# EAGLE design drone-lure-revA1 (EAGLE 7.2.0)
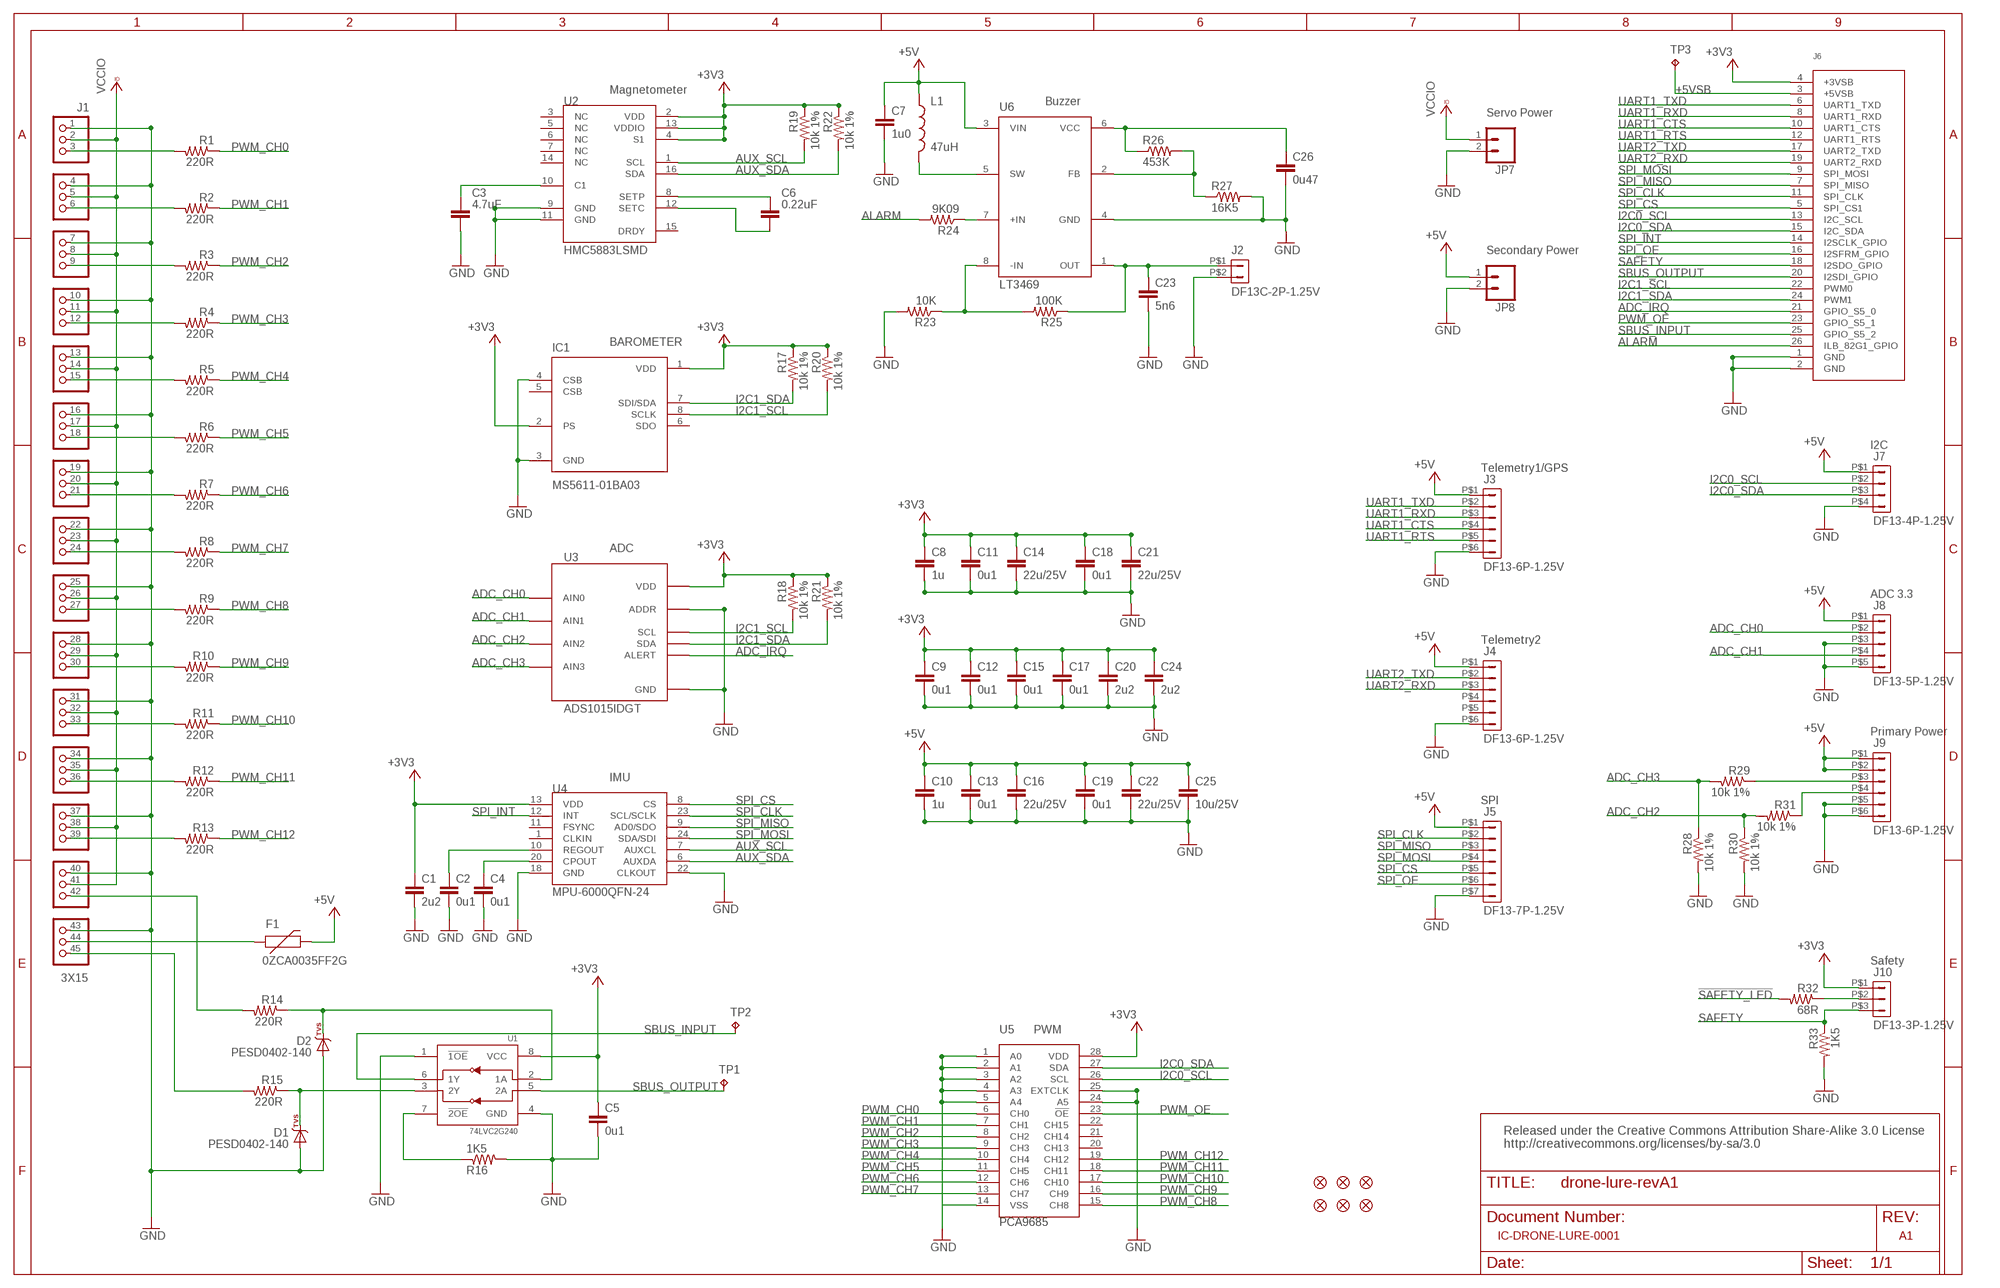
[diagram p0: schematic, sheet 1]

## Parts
C1  2u2  CAP0603  [0603-CAP]
C2  0u1  CAP0402  [0402-CAP]
C3  4.7uF  CAPACITOR_NPOL-0805  [C805]
C4  0u1  CAP0402  [0402-CAP]
C5  0u1  CAP0402  [0402-CAP]
C6  0.22uF  CAPACITOR_NPOL-0805  [C805]
C7  1u0  CAP0603  [0603-CAP]
C8  1u  CAP0603  [0603-CAP]
C9  0u1  CAP0402  [0402-CAP]
C10  1u  CAP0603  [0603-CAP]
C11  0u1  CAP0402  [0402-CAP]
C12  0u1  CAP0402  [0402-CAP]
C13  0u1  CAP0402  [0402-CAP]
C14  22u/25V  CAP0805  [0805-CAP]
C15  0u1  CAP0402  [0402-CAP]
C16  22u/25V  CAP0805  [0805-CAP]
C17  0u1  CAP0402  [0402-CAP]
C18  0u1  CAP0402  [0402-CAP]
C19  0u1  CAP0402  [0402-CAP]
C20  2u2  CAP0603  [0603-CAP]
C21  22u/25V  CAP0805  [0805-CAP]
C22  22u/25V  CAP0805  [0805-CAP]
C23  5n6  CAP0402  [0402-CAP]
C24  2u2  CAP0603  [0603-CAP]
C25  10u/25V  CAP0805  [0805-CAP]
C26  0u47  CAP0402  [0402-CAP]
D1  PESD0402-140  DIODE-TVS  [0402-TVS]
D2  PESD0402-140  DIODE-TVS  [0402-TVS]
F1  0ZCA0035FF2G  PTCSMD  [PTC-1206]
IC1  MS5611-01BA03  [SON125P300X500X100-8N]
J1  3X15  [3X15]
J2  DF13C-2P-1.25V  DF13-2P-1.25V  [DF13C-2P-1.25V]
J3  DF13-6P-1.25V  [DF13C-6P-1.25V]
J4  DF13-6P-1.25V  [DF13C-6P-1.25V]
J5  DF13-7P-1.25V  [DF13C-7P-1.25V]
J6  MBM_LOW_SPEED  [MBM_LOW_SPEED]
J7  DF13-4P-1.25V  [DF13C-4P-1.25V]
J8  DF13-5P-1.25V  [DF13C-5P-1.25V]
J9  DF13-6P-1.25V  [DF13C-6P-1.25V]
J10  DF13-3P-1.25V  [DF13C-3P-1.25V]
JP1  FIDUCIAL1X2.5  [FIDUCIAL-1X2.5]
JP2  FIDUCIAL1X2.5  [FIDUCIAL-1X2.5]
JP3  FIDUCIAL1X2.5  [FIDUCIAL-1X2.5]
JP4  FIDUCIAL1X2.5  [FIDUCIAL-1X2.5]
JP5  FIDUCIAL1X2.5  [FIDUCIAL-1X2.5]
JP6  FIDUCIAL1X2.5  [FIDUCIAL-1X2.5]
JP7  M023.5MM  [SCREWTERMINAL-3.5MM-2]
JP8  M023.5MM  [SCREWTERMINAL-3.5MM-2]
L1  47uH  INDUCTOR0805  [0805-IND]
R1  220R  RESISTOR0402-RES  [0402-RES]
R2  220R  RESISTOR0402-RES  [0402-RES]
R3  220R  RESISTOR0402-RES  [0402-RES]
R4  220R  RESISTOR0402-RES  [0402-RES]
R5  220R  RESISTOR0402-RES  [0402-RES]
R6  220R  RESISTOR0402-RES  [0402-RES]
R7  220R  RESISTOR0402-RES  [0402-RES]
R8  220R  RESISTOR0402-RES  [0402-RES]
R9  220R  RESISTOR0402-RES  [0402-RES]
R10  220R  RESISTOR0402-RES  [0402-RES]
R11  220R  RESISTOR0402-RES  [0402-RES]
R12  220R  RESISTOR0402-RES  [0402-RES]
R13  220R  RESISTOR0402-RES  [0402-RES]
R14  220R  RESISTOR0402-RES  [0402-RES]
R15  220R  RESISTOR0402-RES  [0402-RES]
R16  1K5  RESISTOR0402-RES  [0402-RES]
R17  10k 1%  RESISTOR0402-RES  [0402-RES]
R18  10k 1%  RESISTOR0402-RES  [0402-RES]
R19  10k 1%  RESISTOR0402-RES  [0402-RES]
R20  10k 1%  RESISTOR0402-RES  [0402-RES]
R21  10k 1%  RESISTOR0402-RES  [0402-RES]
R22  10k 1%  RESISTOR0402-RES  [0402-RES]
R23  10K  RESISTOR0402-RES  [0402-RES]
R24  9K09  RESISTOR0402-RES  [0402-RES]
R25  100K  RESISTOR0402-RES  [0402-RES]
R26  453K  RESISTOR0402-RES  [0402-RES]
R27  16K5  RESISTOR0402-RES  [0402-RES]
R28  10k 1%  RESISTOR0402-RES  [0402-RES]
R29  10k 1%  RESISTOR0402-RES  [0402-RES]
R30  10k 1%  RESISTOR0402-RES  [0402-RES]
R31  10k 1%  RESISTOR0402-RES  [0402-RES]
R32  68R  RESISTOR0402-RES  [0402-RES]
R33  1K5  RESISTOR0402-RES  [0402-RES]
TP1  TPTP07SQ  [TP07SQ]
TP2  TPTP07SQ  [TP07SQ]
TP3  TPTP15SQ  [TP15SQ]
U1  74LVC2G240  74LVC2G240-TSSOP-8  [TSSOP8_SOT505-2]
U2  HMC5883LSMD  [16LPCC]
U3  ADS1015IDGT  [MSOP10_0.5]
U4  MPU-6000QFN-24  [QFN-24-TESTING]
U5  PCA9685  [TSSOP-28_4MM]
U6  LT3469  [SOT23-8]

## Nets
!SAFETY_LED: R32.P$2
!SBUS_OUTPUT_EN: R16.P$1 U1.7(!2OE)
+3V3 [power]: C1.P$1 C5.P$1 C8.P$1 C9.P$1 C11.P$1 C12.P$1 C14.P$1 C15.P$1 C17.P$1 C18.P$1 C20.P$1 C21.P$1 C24.P$1 IC1.1(VDD) IC1.2(PS) J6.4(+3VSB) J10.P$1 R17.P$1 R18.P$1 R19.P$1 R20.P$1 R21.P$1 R22.P$1 U1.8(VCC) U2.2(VDD) U2.4(S1) U2.13(VDDIO) U3.8(VDD) U4.13(VDD) U5.28(VDD)
+5V [power]: C7.P$1 C10.P$1 C13.P$1 C16.P$1 C19.P$1 C22.P$1 C25.P$1 F1.2 J3.P$1 J4.P$1 J5.P$1 J7.P$1 J8.P$1 J9.P$1 J9.P$2 JP8.1 L1.P$1 U6.3(VIN)
+5VSB: J6.3(+5VSB) TP3.TP
ADC_CH0: J8.P$2 U3.4(AIN0)
ADC_CH1: J8.P$4 U3.5(AIN1)
ADC_CH2: R30.P$1 R31.P$2 U3.6(AIN2)
ADC_CH3: R28.P$1 R29.P$2 U3.7(AIN3)
ADC_IRQ: J6.21(GPIO_S5_0) U3.2(ALERT)
ALARM: J6.26(ILB_82G1_GPIO) R24.P$2
AUX_SCL: R19.P$2 U2.1(SCL) U4.7(AUXCL)
AUX_SDA: R22.P$2 U2.16(SDA) U4.6(AUXDA)
GND [power]: C1.P$2 C2.P$2 C3.2 C4.P$2 C5.P$2 C7.P$2 C8.P$2 C9.P$2 C10.P$2 C11.P$2 C12.P$2 C13.P$2 C14.P$2 C15.P$2 C16.P$2 C17.P$2 C18.P$2 C19.P$2 C20.P$2 C21.P$2 C22.P$2 C23.P$2 C24.P$2 C25.P$2 C26.P$2 D1.A D2.A IC1.3(GND) IC1.4(CSB) J1.1 J1.4 J1.7 J1.10 J1.13 J1.16 J1.19 J1.22 J1.25 J1.28 J1.31 J1.34 J1.37 J1.40 J1.43 J2.P$2 J3.P$6 J4.P$6 J5.P$7 J6.1(GND) J6.2(GND) J7.P$4 J8.P$3 J8.P$5 J9.P$5 J9.P$6 JP7.2 JP8.2 R16.P$2 R23.P$2 R27.P$2 R28.P$2 R30.P$2 R33.P$2 U1.1(!1OE) U1.4(GND) U2.9(GND) U2.11(GND) U3.1(ADDR) U3.3(GND) U4.18(GND) U4.22(CLKOUT) U5.1(A0) U5.2(A1) U5.3(A2) U5.4(A3) U5.5(A4) U5.14(VSS) U5.24(A5) U5.25(EXTCLK) U6.4(GND)
I2C0_SCL: J6.13(I2C_SCL) J7.P$2 U5.26(SCL)
I2C0_SDA: J6.15(I2C_SDA) J7.P$3 U5.27(SDA)
I2C1_SCL: IC1.8(SCLK) J6.22(PWM0) R18.P$2 R20.P$2 U3.10(SCL)
I2C1_SDA: IC1.7(SDI/SDA) J6.24(PWM1) R17.P$2 R21.P$2 U3.9(SDA)
N$1: C3.1 U2.10(C1)
N$2: J10.P$2 R32.P$1
N$3: C6.1 U2.8(SETP)
N$4: C6.2 U2.12(SETC)
N$5: J9.P$3 R29.P$1
N$6 [power]: F1.1 J1.44
N$7: J9.P$4 R31.P$1
N$8: J1.39 R13.P$2
N$9: J1.36 R12.P$2
N$10: J1.33 R11.P$2
N$11: J1.30 R10.P$2
N$12: J1.27 R9.P$2
N$13: J1.24 R8.P$2
N$14: J1.21 R7.P$2
N$15: J1.18 R6.P$2
N$16: J1.15 R5.P$2
N$17: J1.12 R4.P$2
N$18: J1.9 R3.P$2
N$19: J1.6 R2.P$2
N$20: J1.3 R1.P$2
N$21: R23.P$1 R25.P$2 U6.8(-IN)
N$23: C2.P$1 U4.10(REGOUT)
N$24: R26.P$2 R27.P$1 U6.2(FB)
N$25: C4.P$1 U4.20(CPOUT)
N$27 [power]: C23.P$1 J2.P$1 R25.P$1 U6.1(OUT)
N$28: R24.P$1 U6.7(+IN)
N$32: L1.P$2 U6.5(SW)
N$36 [power]: C26.P$1 R26.P$1 U6.6(VCC)
N$38: D1.C R15.P$1 U1.3(2Y)
PPM-SBUS-PROT [power]: J1.42 R14.P$2
PPM_INPUT: D2.C R14.P$1 U1.2(1A)
PWM_CH0: R1.P$1 U5.6(CH0)
PWM_CH1: R2.P$1 U5.7(CH1)
PWM_CH2: R3.P$1 U5.8(CH2)
PWM_CH3: R4.P$1 U5.9(CH3)
PWM_CH4: R5.P$1 U5.10(CH4)
PWM_CH5: R6.P$1 U5.11(CH5)
PWM_CH6: R7.P$1 U5.12(CH6)
PWM_CH7: R8.P$1 U5.13(CH7)
PWM_CH8: R9.P$1 U5.15(CH8)
PWM_CH9: R10.P$1 U5.16(CH9)
PWM_CH10: R11.P$1 U5.17(CH10)
PWM_CH11: R12.P$1 U5.18(CH11)
PWM_CH12: R13.P$1 U5.19(CH12)
PWM_OE: J6.23(GPIO_S5_1) U5.23(!OE)
SAFETY: J6.18(I2SDO_GPIO) J10.P$3 R33.P$1
SB [power]: J1.45 R15.P$2
SBUS_INPUT: J6.25(GPIO_S5_2) TP2.TP U1.6(1Y)
SBUS_OUTPUT: J6.20(I2SDI_GPIO) TP1.TP U1.5(2A)
SPI_CLK: J5.P$2 J6.11(SPI_CLK) U4.23(SCL/SCLK)
SPI_CS: J5.P$5 J6.5(SPI_CS1) U4.8(CS)
SPI_INT: J6.14(I2SCLK_GPIO) U4.12(INT)
SPI_MISO: J5.P$3 J6.7(SPI_MISO) U4.9(AD0/SDO)
SPI_MOSI: J5.P$4 J6.9(SPI_MOSI) U4.24(SDA/SDI)
SPI_OE: J5.P$6 J6.16(I2SFRM_GPIO)
UART1_CTS: J3.P$4 J6.10(UART1_CTS)
UART1_RTS: J3.P$5 J6.12(UART1_RTS)
UART1_RXD: J3.P$3 J6.8(UART1_RXD)
UART1_TXD: J3.P$2 J6.6(UART1_TXD)
UART2_RXD: J4.P$3 J6.19(UART2_RXD)
UART2_TXD: J4.P$2 J6.17(UART2_TXD)
VCCIO [power]: J1.2 J1.5 J1.8 J1.11 J1.14 J1.17 J1.20 J1.23 J1.26 J1.29 J1.32 J1.35 J1.38 J1.41 JP7.1
Unconnected: IC1.5(CSB) IC1.6(SDO) J4.P$4 J4.P$5 U2.3(NC) U2.5(NC) U2.6(NC) U2.7(NC) U2.14(NC) U2.15(DRDY) U4.1(CLKIN) U4.11(FSYNC) U5.20(CH13) U5.21(CH14) U5.22(CH15)

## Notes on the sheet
- Magnetometer
- Buzzer
- Servo Power
- Secondary Power
- BAROMETER
- I2C
- Telemetry1/GPS
- ADC
- ADC 3.3
- Telemetry2
- Primary Power
- IMU
- SPI
- Safety
- PWM
- Released under the Creative Commons Attribution Share-Alike 3.0 License
  http://creativecommons.org/licenses/by-sa/3.0
- IC-DRONE-LURE-0001 | A1

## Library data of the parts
C1 C2 C4 C5 C9 C11-C13 C15 C17-C19 = pixhawk2:CAP: Capacitor; PARTNO: CC0402ZRY5V7BB104
C3 C6 = dp_devices:CAPACITOR_NPOL: Non-Polarized capacitor in various packages
C7 C8 C10 = pixhawk2:CAP: Capacitor; PARTNO: CC0603ZRY5V7BB105
C14 C16 C21 C22 C25 = pixhawk2:CAP: Capacitor; PARTNO: CL21A226MAQNNNE
C20 C24 = pixhawk2:CAP: Capacitor; PARTNO: C1608Y5V1C225Z
C23 = pixhawk2:CAP: Capacitor; PARTNO: CC0402KRX7R7BB562
C26 = pixhawk2:CAP: Capacitor; PARTNO: C1005X5R1C474K050BC
D1 D2 = pixhawk2:DIODE-TVS; PARTNO: PESD0402-140
F1 = pixhawk2:PTC: Resettable Fuse PTC; PARTNO: 0ZCA0035FF2G
IC1 = Measurement-Specialties:MS5611-01BA03: Variometer Module, with stainless steel cap
J1 = micro-lse-lure:3X15
J2 = con-hirose-df13:DF13-2P-1.25: DF13-2P; PARTNO: DF13C-2P-1.25V(20)
J3 J4 J9 = con-hirose-df13:DF13-6P-1.25: DF13-6P 1.25mm Pitch Miniature Crimping Connector.
J5 = con-hirose-df13:DF13-7P-1.25: DF13-7P 1.25mm Pitch Miniature Crimping Connector.
J6 = micro-lse-lure:MBM_LOW_SPEED; MANEX: 235-0005475
J7 = con-hirose-df13:DF13-4P-1.25: DF13-4P 1.25mm Pitch Miniature Crimping Connector.
J8 = con-hirose-df13:DF13-5P-1.25: DF13-5P 1.25mm Pitch Miniature Crimping Connector.
J10 = con-hirose-df13:DF13-3P-1.25: DF13-3P 1.25mm Pitch Miniature Crimping Connector.
JP1-JP6 = pixhawk2:FIDUCIAL: Fiducial Alignment Points
JP7 JP8 = SparkFun-Connectors:M02: Standard 2-pin 0.1" header. Use with; PROD_ID: CONN-08399
L1 = pixhawk2:INDUCTOR: Inductors; PARTNO: MLZ2012M470W
R1-R22 R28-R33 = pixhawk2:RESISTOR: Resistor; PARTNO: RC0402FR-07220RL
R23 = pixhawk2:RESISTOR: Resistor; PARTNO: RC0402FR-0710KL
R24 = pixhawk2:RESISTOR: Resistor; PARTNO: RMCF0402FT9K09
R25 = pixhawk2:RESISTOR: Resistor; PARTNO: RC0402FR-07100KL
R26 = pixhawk2:RESISTOR: Resistor; PARTNO: RMCF0402FT453K
R27 = pixhawk2:RESISTOR: Resistor; PARTNO: RMCF0402FT16K5
TP1-TP3 = testpad:TP: Test pad
U1 = pixhawk2:74LVC2G240: Dual inverter tri-state, 3.3V/5V compatible http://www.nxp.com/documents/data_sheet/74LVC2G240.pdf http://focus.ti.com/lit/ds/symlink/sn74lvc2g240.pdf; PARTNO: 74LVC2G240DP,125
U2 = SparkFun-Sensors:HMC5883L: 3 Axis Digital Compass IC
U3 = bt_adc:ADS1015: Ti ADS1015 12-bit ADC Ultra-Small, Low-Power, 12-Bit Analog-to-Digital Converter with Internal Reference The ADS1013, ADS1014, and ADS1015 are precision analog-to-digital converters (ADCs) with 12 bits of resolution offered in an ultra-small, leadless QFN-10 package or an MSOP-10 package. \ Source: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
U4 = SparkFun-Sensors:MPU-6000: MPU-6000 - I2C address is 0x68 with AD0 low and 0x69 with AD0 high.
U5 = SparkFun-DigitalIC:PCA9685: 16-channel 12-bit PWM I2C interface Internal Oscillator 40Hz to 1kHz Can be totem pole or open collector 2.3V to 5.5V; PROD_ID: IC-12240
U6 = pixhawk2:LT3469: LT3469 Piezo microactuator driver with boost regulator; PARTNO: LT3469ETS8

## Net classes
0 default: width 0.254 mm, drill 0.305 mm, clearance 0.152 mm
1 power: width 0.508 mm, drill 0.305 mm, clearance 0.254 mm

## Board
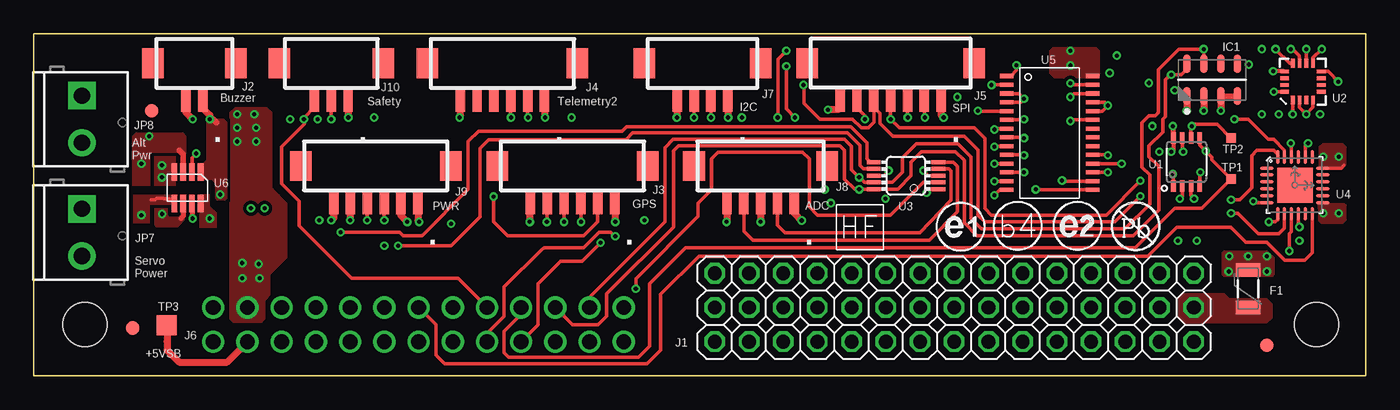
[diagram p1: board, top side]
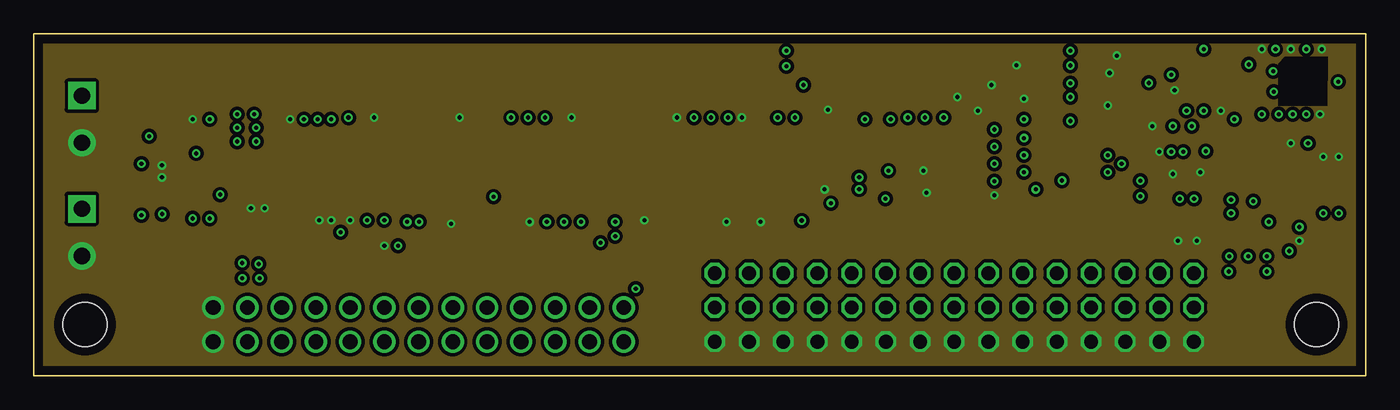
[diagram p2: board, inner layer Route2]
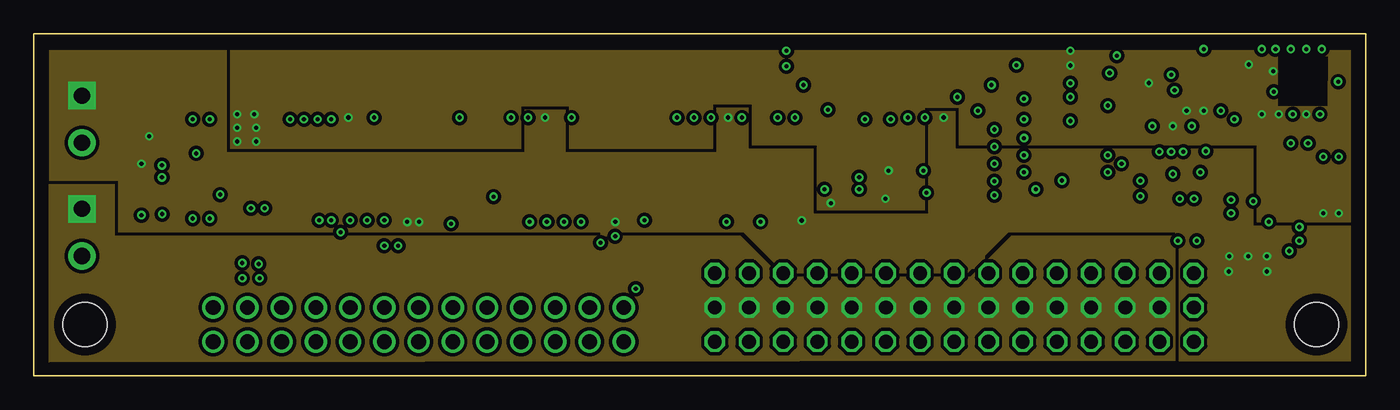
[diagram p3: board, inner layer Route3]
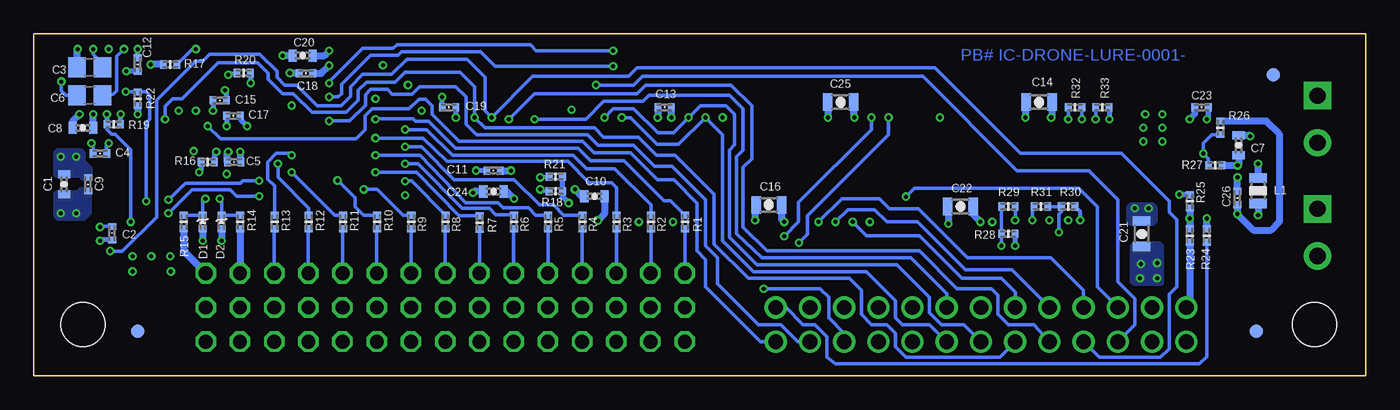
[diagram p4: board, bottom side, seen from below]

Size 98.91 x 25.4 mm. Coordinates in mm from the lower left corner, seen from the top.
Copper layers (1+2*3+16): Top 0.01714375mm / dielectric 0.09398125mm / Route2 0.034290625mm / dielectric 49mil / Route3 0.034290625mm / dielectric 0.09398125mm / Bottom 0.01714375mm
Design rules "default *": minimum track width 5mil, minimum drill 10mil, track to track 6mil, track to pad 6mil, pad to pad 15mil, via to via 10mil, smd to smd 5mil, copper to edge 25mil, drill to drill 10mil, minimum pad ring 10mil, minimum via ring 6mil, stop-mask expansion 2.5mil, vias tented up to drill 20mil, thermal gap 10mil
tRestrict: area 50.9,13.9 to 57.1,16.3; 4 lines
bRestrict: 4 lines
vRestrict: 4 lines

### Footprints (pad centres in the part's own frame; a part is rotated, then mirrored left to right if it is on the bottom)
0603-CAP = smd 0.6 x 0.9: P$1 -0.75,0; P$2 0.75,0
0402-CAP = smd 0.5 x 0.6: P$1 -0.5,0; P$2 0.5,0
C805 = smd 1.3 x 1.5: 1 -0.95,0; 2 0.95,0
0805-CAP = smd 0.7 x 1.3: P$1 -0.95,0; P$2 0.95,0
0402-TVS = smd 0.5 x 0.6: A 0.5,0; C -0.5,0
PTC-1206 = smd 1 x 1.8: 1 -1.4,0; 2 1.4,0
SON125P300X500X100-8N = smd 1.35 x 0.55: 1 -1.2,1.875; 2 -1.2,0.625; 3 -1.2,-0.625; 4 -1.2,-1.875; 5 1.2,-1.875; 6 1.2,-0.625; 7 1.2,0.625; 8 1.2,1.875
3X15 = drill 1.016 octagon: 1 -19.05,-2.54; 2 -19.05,0; 3 -19.05,2.54; 4 -16.51,-2.54; 5 -16.51,0; 6 -16.51,2.54; 7 -13.97,-2.54; 8 -13.97,0; 9 -13.97,2.54; 10 -11.43,-2.54; 11 -11.43,0; 12 -11.43,2.54; 13 -8.89,-2.54; 14 -8.89,0; 15 -8.89,2.54; 16 -6.35,-2.54; 17 -6.35,0; 18 -6.35,2.54; 19 -3.81,-2.54; 20 -3.81,0; 21 -3.81,2.54; 22 -1.27,-2.54; 23 -1.27,0; 24 -1.27,2.54; 25 1.27,-2.54; 26 1.27,0; 27 1.27,2.54; 28 3.81,-2.54; 29 3.81,0; 30 3.81,2.54; 31 6.35,-2.54; 32 6.35,0; 33 6.35,2.54; 34 8.89,-2.54; 35 8.89,0; 36 8.89,2.54; 37 11.43,-2.54; 38 11.43,0; 39 11.43,2.54; 40 13.97,-2.54; 41 13.97,0; 42 13.97,2.54; 43 16.51,-2.54; 44 16.51,0; 45 16.51,2.54
DF13C-2P-1.25V = smd 1.6 x 2.2: M$0 3.075,-1.8; M$1 -3.075,-1.8 | smd 0.7 x 1.8: P$1 -0.625,0.9; P$2 0.625,0.9
DF13C-6P-1.25V = smd 1.6 x 2.2: M$0 5.575,-1.8; M$1 -5.575,-1.8 | smd 0.7 x 1.8: P$1 -3.125,0.9; P$2 -1.875,0.9; P$3 -0.625,0.9; P$4 0.625,0.9; P$5 1.875,0.9; P$6 3.125,0.9
DF13C-7P-1.25V = smd 1.6 x 2.2: M$0 6.2,-1.8; M$1 -6.2,-1.8 | smd 0.7 x 1.8: P$1 -3.75,0.9; P$2 -2.5,0.9; P$3 -1.25,0.9; P$4 0,0.9; P$5 1.25,0.9; P$6 2.5,0.9; P$7 3.75,0.9
MBM_LOW_SPEED = drill 1.1: 1 -15.24,0; 2 -15.24,2.54; 3 -12.7,0; 4 -12.7,2.54; 5 -10.16,0; 6 -10.16,2.54; 7 -7.62,0; 8 -7.62,2.54; 9 -5.08,0; 10 -5.08,2.54; 11 -2.54,0; 12 -2.54,2.54; 13 0,0; 14 0,2.54; 15 2.54,0; 16 2.54,2.54; 17 5.08,0; 18 5.08,2.54; 19 7.62,0; 20 7.62,2.54; 21 10.16,0; 22 10.16,2.54; 23 12.7,0; 24 12.7,2.54; 25 15.24,0; 26 15.24,2.54 | hole 3.302: -24.765,1.27; 66.675,1.27
DF13C-4P-1.25V = smd 1.6 x 2.2: M$0 4.325,-1.8; M$1 -4.325,-1.8 | smd 0.7 x 1.8: P$1 -1.875,0.9; P$2 -0.625,0.9; P$3 0.625,0.9; P$4 1.875,0.9
DF13C-5P-1.25V = smd 1.6 x 2.2: M$0 4.95,-1.8; M$1 -4.95,-1.8 | smd 0.7 x 1.8: P$1 -2.5,0.9; P$2 -1.25,0.9; P$3 0,0.9; P$4 1.25,0.9; P$5 2.5,0.9
DF13C-3P-1.25V = smd 1.6 x 2.2: M$0 3.85,-1.8; M$1 -3.85,-1.8 | smd 0.7 x 1.8: P$1 -1.25,0.9; P$2 0,0.9; P$3 1.25,0.9
FIDUCIAL-1X2.5 = smd 1 x 1: 1 0,0
SCREWTERMINAL-3.5MM-2 = drill 1.2 pad 2.032 square: 1 0,0 | drill 1.2 pad 2.032: 2 3.5,0
0805-IND = smd 0.7 x 1.3: P$1 -0.95,0; P$2 0.95,0
0402-RES = smd 0.5 x 0.6: P$1 -0.5,0; P$2 0.5,0
TP07SQ = smd 0.7 x 0.7: TP 0,0
TP15SQ = smd 1.5 x 1.5: TP 0,0
TSSOP8_SOT505-2 = smd 0.35 x 0.85: 1 -0.975,-1.775; 2 -0.325,-1.775; 3 0.325,-1.775; 4 0.975,-1.775; 5 0.975,1.775; 6 0.325,1.775; 7 -0.325,1.775; 8 -0.975,1.775
16LPCC = smd 0.65 x 0.28: 1 -1.37,0.75; 2 -1.37,0.25; 3 -1.37,-0.25; 4 -1.37,-0.75; 9 1.37,-0.75; 10 1.37,-0.25; 11 1.37,0.25; 12 1.37,0.75 | smd 0.28 x 0.65: 5 -0.75,-1.37; 6 -0.25,-1.37; 7 0.25,-1.37; 8 0.75,-1.37; 13 0.75,1.37; 14 0.25,1.37; 15 -0.25,1.37; 16 -0.75,1.37
MSOP10_0.5 = smd 0.3 x 1.02: 1 -1,-2.4; 2 -0.5,-2.4; 3 0,-2.4; 4 0.5,-2.4; 5 1,-2.4; 6 1,2.4; 7 0.5,2.4; 8 0,2.4; 9 -0.5,2.4; 10 -1,2.4
QFN-24-TESTING = smd 1.016 x 0.254: 1 -2.066,1.257; 2 -2.066,0.75; 3 -2.066,0.247; 4 -2.066,-0.287; 5 -2.066,-0.792; 6 -2.066,-1.297; 13 2.086,-1.297; 14 2.086,-0.792; 15 2.086,-0.287; 16 2.086,0.247; 17 2.086,0.75; 18 2.086,1.257 | smd 0.254 x 1.016: 7 -1.267,-2.122; 8 -0.762,-2.122; 9 -0.258,-2.122; 10 0.278,-2.122; 11 0.78,-2.122; 12 1.287,-2.122; 19 1.287,2.082; 20 0.78,2.082; 21 0.278,2.082; 22 -0.258,2.082; 23 -0.762,2.082; 24 -1.267,2.082 | smd 2.616 x 2.616: P$1 0.02,-0.01
TSSOP-28_4MM = smd 1 x 0.3: 1 -3.2,4.225; 2 -3.2,3.575; 3 -3.2,2.925; 4 -3.2,2.275; 5 -3.2,1.625; 6 -3.2,0.975; 7 -3.2,0.325; 8 -3.2,-0.325; 9 -3.2,-0.975; 10 -3.2,-1.625; 11 -3.2,-2.275; 12 -3.2,-2.925; 13 -3.2,-3.575; 14 -3.2,-4.225; 15 3.2,-4.225; 16 3.2,-3.575; 17 3.2,-2.925; 18 3.2,-2.275; 19 3.2,-1.625; 20 3.2,-0.975; 21 3.2,-0.325; 22 3.2,0.325; 23 3.2,0.975; 24 3.2,1.625; 25 3.2,2.275; 26 3.2,2.925; 27 3.2,3.575; 28 3.2,4.225
SOT23-8 = smd 0.42 x 1.3: 1 -0.975,-1.175; 2 -0.325,-1.175; 3 0.325,-1.175; 4 0.975,-1.175; 5 0.975,1.175; 6 0.325,1.175; 7 -0.325,1.175; 8 -0.975,1.175

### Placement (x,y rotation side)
C1  96.65,14.22 90 bottom
C2  93.09,10.59 270 bottom
C3  94.74,22.91 180 bottom
C4  93.98,16.51 0 bottom
C5  84.02,15.88 0 bottom
C6  94.74,20.83 0 bottom
C7  9.45,17.12 270 bottom
C8  95.25,18.41 180 bottom
C9  94.87,14.22 90 bottom
C10  57.28,13.34 180 bottom
C11  64.77,15.24 180 bottom
C12  91.19,23.11 90 bottom
C13  52.07,19.94 180 bottom
C14  24.26,20.32 180 bottom
C15  85.09,20.45 0 bottom
C16  44.32,12.7 180 bottom
C17  84.07,19.3 0 bottom
C18  78.69,22.45 180 bottom
C19  68.07,19.94 180 bottom
C20  78.94,23.77 180 bottom
C21  16.64,10.54 90 bottom
C22  30.1,12.57 180 bottom
C23  12.19,19.94 0 bottom
C24  64.77,13.69 180 bottom
C25  38.99,20.32 180 bottom
C26  9.55,13.21 90 bottom
D1  86.36,11.43 270 bottom
D2  84.96,11.43 270 bottom
DRILEGEND  [DRILEGEND]  not placed on the board
F1  90.17,6.48 90 top
IC1  87.5,21.97 90 top
J1  69.62,5.08 0 top
J2  11.94,21.41 180 top
J3  40.01,13.79 180 top
J4  34.8,21.41 180 top
J5  63.63,21.41 180 top
J6  28.57,2.54 0 top
J7  49.66,21.41 180 top
J8  53.98,13.79 180 top
J9  25.4,13.79 180 top
J10  22.1,21.41 180 top
JP1  7.37,3.56 90 top
JP2  8.13,3.3 90 bottom
JP3  8.76,19.68 90 top
JP4  6.86,22.35 90 bottom
JP5  91.57,2.29 90 top
JP6  91.19,3.3 90 bottom
JP7  3.58,12.4 270 top
JP8  3.58,20.81 270 top
L1  8,13.74 270 bottom
R1  50.55,11.43 270 bottom
R2  53.09,11.43 270 bottom
R3  55.63,11.43 270 bottom
R4  58.17,11.43 270 bottom
R5  60.71,11.43 270 bottom
R6  63.25,11.43 270 bottom
R7  65.79,11.38 270 bottom
R8  68.33,11.43 270 bottom
R9  70.87,11.43 270 bottom
R10  73.41,11.43 270 bottom
R11  75.95,11.43 270 bottom
R12  78.49,11.43 270 bottom
R13  81.03,11.43 270 bottom
R14  83.57,11.43 270 bottom
R15  87.76,11.43 270 bottom
R16  85.98,15.88 180 bottom
R17  88.77,23.11 0 bottom
R18  60.15,13.72 180 bottom
R19  92.96,18.67 180 bottom
R20  83.31,22.48 180 bottom
R21  60.15,14.78 180 bottom
R22  91.19,20.57 90 bottom
R23  13.08,10.41 270 bottom
R24  11.81,10.41 270 bottom
R25  13.08,12.95 270 bottom
R26  10.79,18.41 270 bottom
R27  11.18,15.62 0 bottom
R28  26.54,10.54 0 bottom
R29  26.54,12.57 180 bottom
R30  22.1,12.57 0 bottom
R31  24.13,12.57 0 bottom
R32  21.59,19.94 0 bottom
R33  19.56,19.94 0 bottom
TP1  88.9,14.61 90 top
TP2  88.9,17.65 90 top
TP3  9.88,3.76 90 top
U1  85.6,15.88 0 top
U2  94.23,21.84 90 top
U3  64.77,14.86 90 top
U4  93.63,14.16 0 top
U5  75.44,18.03 0 top
U6  11.43,13.97 180 top

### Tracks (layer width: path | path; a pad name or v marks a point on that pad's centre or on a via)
!SAFETY_LED  (via drill 0.3)
  Bottom 0.254: R32.P$2 21.09,19.18 v21.08,19.05
!SBUS_OUTPUT_EN  (via drill 0.3)
  Top 0.254: U1.7 85.27,16.69 v85.34,16.64
  Bottom 0.381: R16.P$1 85.48,16.5 v85.34,16.64
+3V3  (via drill 0.3)
  Top 0.254: U2.2 93.98,19.93 v94.49,19.43 94.98,19.93 U2.4 | U3.8 63.12,14.86 63.32,15.06 v63.48,15.24
  Top 0.305: U1.8 84.62,16.8 v84.45,16.64 | U2.13 92.09,22.59 v92.02,22.61
  Top 0.356: U1.8 84.62,18.5 v84.58,18.54
  Top 0.508: 85.6,20.74 IC1.1 85.63,19.71 v85.6,19.68 | IC1.2 86.88,19.7 v86.87,19.68 | 23.37,20.48 J10.P$1 23.35,19.2 v23.37,19.18
  Bottom 0.381: C15.P$1 85.59,19.69 | C12.P$1 92.07,22.61 | v92.46,19.43 v92.46,19.42 R19.P$1 | 84.52,16.55 v84.45,16.64 | C17.P$1 v84.57,18.55 v84.58,18.54 | R20.P$1 82.8,22.34 v82.8,21.74 | v59.18,12.83 59.65,13.29 R18.P$1 R21.P$1
  Bottom 0.508: 85.59,19.69 v85.6,19.68 | v84.57,18.53 v84.58,18.54 | 92.07,22.61 v92.02,22.61 | R22.P$1 91.18,19.57 v91.19,19.43 | v94.5,19.42 v94.49,19.43 94.49,19.3 C8.P$1 | C11.P$1 v63.48,15.24 | C14.P$1 23.31,19.24 v23.37,19.18 | R17.P$1 v90.22,23.11 | C20.P$1 77.32,23.77 v76.96,24.13 | C18.P$1 77.55,22.45 v76.96,23.04 | C24.P$1 63.78,13.69 v63.25,13.16 | C5.P$1 84.52,16.57 v84.45,16.64
  other vias: 95.76,12.06 96.9,12.06 16.71,8.31 15.49,8.38 15.49,7.24 16.76,7.24 15.11,19.43 16.38,19.43 16.51,17.4 15.11,17.4 16.51,18.41 15.11,18.41
  pour Top (no thermals): 78.99,22.1 75.82,22.1 75.44,22.48 75.44,24 75.44,24.13 75.69,24.38 78.87,24.38 79.12,24.13 79.12,22.23
  pour Top (no thermals): 75.82,22.1 75.44,22.48 75.44,24.13 75.69,24.38 78.87,24.38 79.12,24.13 79.12,22.23 79.06,22.17 77.97,22.17 77.95,22.14 77.54,22.14 77.36,22.32 77.1,22.43 76.82,22.43 76.56,22.32 76.36,22.12 76.35,22.1
  pour Top (rank 2, no thermals): 16.89,3.94 14.86,3.94 14.61,4.19 14.61,19.56 14.99,19.94 17.27,19.94 17.65,19.56 17.65,13.97 18.8,12.83 18.8,8.76 17.53,7.49 17.53,5.97 17.14,5.59 17.14,4.19
  pour Top (no thermals): 97.28,12.83 97.41,12.7 97.41,11.56 97.16,11.3 95.63,11.3 95.38,11.56 95.38,12.83 95.36,12.84 96.06,12.84 96.05,12.83
  pour Top (no thermals): 75.82,22.1 75.44,22.48 75.44,24.13 75.69,24.38 78.87,24.38 79.12,24.13 79.12,22.23 79.06,22.17 77.97,22.17 77.95,22.14 77.54,22.14 77.36,22.32 77.1,22.43 76.82,22.43 76.56,22.32 76.36,22.12 76.35,22.1
  pour Bottom (no thermals): 95.5,13.97 95.76,13.72 97.28,13.72 97.41,13.59 97.41,11.81 97.16,11.56 95.12,11.56 94.61,12.06 94.61,13.97
  pour Route3 (no thermals): 14.61,24.13 14.61,16.89 36.2,16.89 36.2,20.07 39.75,20.07 39.75,16.89 50.42,16.89 50.42,20.19 53.34,20.19 53.34,17.14 58.17,17.14 58.17,12.32 66.17,12.32 66.17,19.94 68.71,19.94 68.71,17.14 90.81,17.14 90.81,11.43 97.79,11.43 97.79,24.13
  pour Bottom (no thermals): 17.27,9.91 17.53,9.65 17.53,6.99 17.27,6.73 15.14,6.73 14.99,6.86 14.99,9.65 15.27,9.91
+5V  (via drill 0.3)
  Top 0.406: U6.3 11.11,16.45 10.79,16.76
  Top 0.508: 28.57,12.84 J9.P$1 28.52,11.53 v28.63,11.43 | v43.18,11.43 43.18,12.84 J3.P$1 | J7.P$1 51.53,19.21 v51.56,19.18 | J4.P$1 37.92,19.23 v37.97,19.18 | J5.P$1 67.38,19.36 v67.56,19.18 | J9.P$2 27.27,11.89 v27.74,11.43 | J8.P$1 56.48,12.08 v57.02,11.53
  Bottom 0.381: C19.P$1 67.57,19.18 v67.56,19.18
  Bottom 0.508: C13.P$1 v51.57,19.18 v51.56,19.18 | C22.P$1 29.13,11.95 v28.63,11.43 | C25.P$1 38.04,19.24 v37.97,19.18 | C16.P$1 43.37,11.62 v43.18,11.43 | 56.52,13.32 C10.P$1 56.53,12.03 v57.02,11.53 | L1.P$1 v8,15.75 | 8.65,17.77 v8.59,17.78 8.68,17.87 C7.P$1
  other vias: 91.57,7.75 91.57,8.89 90.17,8.89 88.77,8.89 88.72,7.75
  pour Top (no thermals): 88.39,7.37 88.27,7.49 88.27,9.14 88.39,9.27 89.78,9.27 89.91,9.27 91.69,9.27 91.95,9.01 92.08,8.89 92.08,7.49 91.95,7.37
  pour Top (no thermals): 11.14,15.96 11.14,14.53 11.07,14.53 11.07,15.96 10.95,16.11 10.95,16.56 8.61,16.56 8.61,14.1 7.37,14.1 7.37,17.78 7.62,18.03 11.05,18.03 11.3,17.78 11.3,16.51 11.22,16.42 11.22,16.05
  pour Route3 (rank 6, no thermals): 97.79,24.13 1.14,24.13 1.14,1.14 97.79,1.14
+5VSB
  Top 0.254: TP3.TP 9.9,3.81 9.99,4.04 9.88,3.89
  Top 0.508: 9.65,3.81 9.9,3.81 9.91,2.54 9.91,1.91 10.79,1.02 14.35,1.02 J6.3
ADC_CH0
  Top 0.254: 55.37,12.74 J8.P$2 55.23,11.17 55.78,10.62 65.79,10.62 68.1,13.06 68.1,15.21 67.95,15.36 U3.4
ADC_CH1
  Top 0.254: J8.P$4 52.73,10.75 53.39,10.08 66.5,10.08 68.58,12.17 68.58,15.57 68.29,15.86 U3.5
ADC_CH2  (via drill 0.3)
  Top 0.254: v22.78,10.67 27.18,10.67 27.43,10.41 28.83,10.41 32.26,13.84 32.26,17.4 33.02,18.16 43.69,18.16 44.02,18.49 60.68,18.49 61.85,17.32 61.85,16.13 62.12,15.86 U3.6
  Bottom 0.254: R31.P$2 R30.P$1 22.6,12.19 22.78,12.01 v22.78,10.67
ADC_CH3  (via drill 0.3)
  Top 0.254: v27.05,9.65 30.99,9.65 33.15,11.81 33.15,16.89 33.78,17.53 43.97,17.53 44.48,18.03 60.43,18.03 61.34,17.12 61.34,15.62 61.6,15.36 U3.7
  Bottom 0.254: R29.P$2 R28.P$1 27.04,9.91 v27.05,9.65
ADC_IRQ  (via drill 0.3)
  Top 0.254: U3.2 66.05,14.36 63.63,11.94 58.19,11.94 57.58,12.55 57.58,16.1 57.07,16.61 50.83,16.61 50.34,16.13 50.34,13.82 49.33,12.8 49.33,11.84 44.7,7.21 v44.7,6.48
  Bottom 0.254: J6.21 38.73,3.17 39.88,4.32 39.88,5.84 40.51,6.48 v44.7,6.48 44.7,6.5
ALARM
  Bottom 0.254: J6.26 43.05,5.08 41.78,3.81 40.89,3.81 40.01,2.92 40.01,1.4 39.4,0.89 12.34,0.89 11.81,1.42 R24.P$2
AUX_SCL  (via drill 0.3)
  Top 0.254: U2.1 93.48,19.57 v93.47,19.43 | U4.7 92.36,11.59 92.2,11.43 v91.69,11.43
  Bottom 0.254: 93.46,19.55 v93.47,19.43 | R19.P$2 93.46,18.28 93.12,17.93 92.84,17.93 91.69,16.79 v91.69,11.43
  Bottom 0.381: R19.P$2 93.46,19.55
AUX_SDA  (via drill 0.3)
  Top 0.254: v90.55,12.95 90.64,12.87 U4.6 | U2.16 92.09,21.09 v92.08,21.08
  Bottom 0.254: R22.P$2 92.07,21.07 v92.08,21.08 | 91.18,21.08 R22.P$2 | v90.55,12.95 90.55,18.8 90.3,19.05 90.3,20.83 90.54,21.07 R22.P$2
GND  (via drill 0.3)
  Top 0.254: 71.27,21.61 v71.12,21.59 71.14,21.61 U5.2 | U5.3 73.16,20.96 v73.53,20.57 73.29,20.31 U5.4 | U1.4 86.57,15.07 v86.61,15.11 | U1.1 84.62,14.92 v84.58,14.99 | U5.25 79.51,20.31 v79.76,20.07 79.35,19.66 U5.24 | U2.11 93.98,23.77 93.5,24.26 v93.34,24.26 | 95,23.21 U2.9 94.98,23.61 v95.63,24.26 | U3.3 66.45,14.86 v66.06,15.24 | U3.1 66.56,13.86 v66.29,13.59 | U5.5 70.13,19.66 v70.1,19.68 | U5.1 72.42,22.26 72.54,22.25 72.97,22.68 v72.97,23.06 | U5.14 71.72,13.81 v71.32,13.41 | U4.22 93.37,17.25 v93.34,17.27 | U4.18 97.08,15.42 97.28,15.62
  Top 0.406: IC1.3 IC1.4
  Top 0.508: J8.P$5 51.48,11.47 v51.44,11.43 | J8.P$3 v53.98,11.43 | J9.P$5 23.5,12.86 v23.5,11.56 | v36.83,11.43 36.83,12.84 J3.P$6 | IC1.3 v88.14,19.68 | J4.P$6 31.67,19.23 v31.62,19.18 | J2.P$2 11.25,20.31 11.25,19.61 v11.81,19.05 | J7.P$4 47.78,19.21 v47.75,19.18 | J5.P$7 59.88,19.9 59.74,19.76 v58.98,19.76 | J9.P$6 22.27,11.73 v22.1,11.56
  Bottom 0.305: v21.21,11.56 21.21,12.18 R30.P$2 | C4.P$2 93.48,17.14 v93.34,17.27
  Bottom 0.381: C2.P$2 93.9,10.09 v93.98,10.03 | C12.P$2 v91.19,24.26 | C4.P$2 | R16.P$2 86.48,15.25 v86.61,15.11 | R33.P$2 19.06,19.18 v19.05,19.05 | 26.04,10.66 R28.P$2 v26.04,9.66 v26.04,9.65 | C19.P$2 v68.57,20.69 v68.58,20.7 | C15.P$2 84.59,21.09 v84.71,21.21 | C11.P$2 v66.06,15.24 | v83.57,16.63 v83.57,16.64 | C17.P$2 83.57,19.06 v83.06,18.54
  Bottom 0.406: C23.P$2 11.69,19.17 v11.81,19.05
  Bottom 0.508: D2.A v84.96,10.03 | D1.A v86.36,10.03 | C13.P$2 v52.57,19.18 v52.58,19.18 | v30.99,11.3 30.99,12.51 C22.P$2 | C3.2 95.69,24.2 v95.63,24.26 | v95.5,19.42 v95.5,19.43 96,18.93 C8.P$2 | C25.P$2 39.94,19.24 39.93,19.24 v39.93,19.18 | C14.P$2 25.27,20.25 v25.27,19.18 | v45.34,11.56 45.34,12.63 C16.P$2 | C26.P$2 9.55,14.71 v9.53,14.73 | C18.P$2 v79.88,22.48 | C20.P$2 v80.42,23.77 | 9.58,15.57 v9.53,15.62 | R27.P$2 v9.53,15.62 | R23.P$2 13.08,5.33 J6.2 | C10.P$2 58.22,13.34 v58.73,13.84 | C24.P$2 66.19,13.69 v66.29,13.59 | C7.P$2 9.45,15.7 v9.53,15.62 | C5.P$2 83.52,16.59 v83.57,16.64
  other vias: 95.76,16.26 96.9,16.26 16.13,12.45 17.14,12.45
  pour Route2 (no thermals): 0,0 98.93,0 98.93,25.4 0,25.4
  pour Route2 (no thermals): 0,0 98.93,0 98.93,25.4 0,25.4
  pour Top (no thermals): 95.45,15.37 95.45,16.99 95.73,17.27 97.16,17.27 97.41,17.02 97.41,15.62 97.16,15.37
  pour Bottom (no thermals): 94.61,14.48 95.25,14.48 95.5,14.73 97.28,14.73 97.41,14.86 97.41,16.64 97.16,16.89 95.38,16.89 95.12,16.64 95.12,16 94.61,15.49
  pour Top (no thermals): 10.52,16.31 10.52,14.12 8.99,14.12 8.99,16.31
  pour Bottom (no thermals): 17.14,11.18 15.75,11.18 15.49,11.43 15.49,12.57 15.75,12.83 16.89,12.83 17.53,12.83 17.78,12.57 17.78,12.06 17.78,11.43 17.53,11.18 17.27,11.18
I2C0_SCL  (via drill 0.3)
  Top 0.254: J7.P$2 v50.28,19.19 v50.29,19.18 | v76.96,20.7 77.21,20.96 U5.26 78.61,20.95 | v55.88,22.99 55.88,19.81 v56.52,19.18
  Bottom 0.254: J6.13 29.84,3.81 31.5,3.81 32.38,4.7 32.38,5.84 34.8,8.26 45.21,8.26 47.24,10.29 47.24,16.76 46.86,17.14 46.86,19.43 47.5,20.07 49.4,20.07 v50.29,19.18 51.41,18.06 52.55,18.06 | v76.96,20.7 76.3,20.7 76.05,20.95 76.05,21.64 73.89,23.8 71.83,23.8 71.58,24.05 65.71,24.05 64.64,22.99 v55.88,22.99 | 52.63,18.14 52.55,18.06 | 52.55,18.06 54.36,19.81 55.88,19.81 v56.52,19.18
I2C0_SDA  (via drill 0.3)
  Top 0.254: J7.P$3 v49.02,19.18 | v76.96,21.72 77.11,21.61 U5.27 78.62,21.59 | v55.24,19.18 55.24,23.5 v55.88,24.13
  Bottom 0.254: J6.15 32.38,3.81 34.42,3.81 34.92,4.32 34.92,5.59 37.08,7.75 45.47,7.75 47.75,10.03 47.75,17.91 v49.02,19.18 | 48.77,18.92 v49.02,19.18 | v76.96,21.72 76.96,21.84 74.5,24.31 72.24,24.31 71.93,24.56 62.03,24.56 61.59,24.13 v55.88,24.13 | v55.24,19.18 54.61,19.18 52.61,17.18 51.02,17.18 v49.02,19.18
I2C1_SCL  (via drill 0.3)
  Top 0.254: 62.38,13.87 U3.10 | 62.36,13.84 U3.10 | U3.10 | IC1.8 85.6,23.14 85.6,22.73 85.22,22.35 v84.45,22.35 84.38,22.35 84.02,22 84.02,19.25 83.82,19.05 83.82,18.09 82.8,17.07 82.8,16.28 83.54,15.54 83.54,12.29 81.66,10.41 70.03,10.41 69.09,11.35 69.09,16 68.45,16.64 65.91,16.64 65.15,15.88 65.15,14.86 64.15,13.86 U3.10 | J6.22 40.01,3.81 41.91,3.81 42.55,4.45 42.55,6.1 47.5,11.05 47.5,16.71 47.88,17.09 59.87,17.09 60.2,16.76 60.2,14.61 60.96,13.84 v61.29,13.84 61.31,13.86 U3.10
  Bottom 0.254: R18.P$2 61.16,13.72 v61.29,13.84 | R20.P$2 84.33,22.48 v84.45,22.35
I2C1_SDA  (via drill 0.3)
  Top 0.254: IC1.7 86.88,24.25 v86.87,24.26 86.84,24.23 85.04,24.23 83.52,22.71 83.52,19.61 83.46,19.51 83.26,19.3 82.8,19.3 82.3,18.8 82.3,15.49 82.86,14.94 82.86,12.75 81.03,10.92 70.36,10.92 69.6,11.68 69.6,16.26 68.63,17.22 65.53,17.22 64.52,16.2 64.52,15.11 63.76,14.36 U3.9 61.66,14.36 v61.29,14.73 60.71,15.32 60.71,17.04 60.2,17.55 47.47,17.55 46.86,16.94 46.86,11.43 41.27,5.84 J6.24
  Bottom 0.254: 86.88,24.25 v86.87,24.26 87.12,24.26 R17.P$2 | R21.P$2 61.24,14.78 v61.29,14.73
N$1  (via drill 0.3)
  Top 0.254: U2.10 v94.48,24.25 v94.49,24.26
  Bottom 0.254: C3.1 93.79,23.18 94.49,23.88 v94.49,24.26
N$2  (via drill 0.3)
  Top 0.254: J10.P$2 v22.1,19.05
  Bottom 0.254: R32.P$1 22.09,19.18 v22.1,19.05
N$3  (via drill 0.3)
  Top 0.254: v96.85,21.84 96.14,22.58 96.13,22.59 U2.8
  Bottom 0.254: C6.1 96.52,20.83 96.85,21.16 v96.85,21.84
N$4  (via drill 0.3)
  Top 0.254: U2.12 93.25,23.21 v92.2,24.26
  Bottom 0.254: C6.2 93.79,20.89 | 93.79,20.89 93.79,21.02 | v92.2,24.26 92.73,23.72 92.73,21.16 93,20.89 93.79,20.89
N$5  (via drill 0.3)
  Top 0.254: v26.04,11.56 26.02,11.57 J9.P$3
  Bottom 0.254: v26.04,11.56 R29.P$1
N$6
  pour Top (no thermals): 91.57,5.71 88.77,5.71 88.39,6.1 85.34,6.1 85.09,5.84 84.84,5.59 84.84,4.95 84.84,4.45 85.34,3.94 90.42,3.94 91.57,3.94 91.95,4.32 91.95,5.33
N$7  (via drill 0.3)
  Top 0.254: J9.P$4 v24.77,11.56
  Bottom 0.254: v24.77,11.56 24.77,12.44 R31.P$1
N$8
  Bottom 0.254: J1.39 81.05,10.9 R13.P$2
N$9
  Bottom 0.254: J1.36 78.51,10.9 R12.P$2
N$10
  Bottom 0.254: J1.33 75.97,10.83 R11.P$2
N$11
  Bottom 0.254: J1.30 73.43,10.9 R10.P$2
N$12
  Bottom 0.254: J1.27 70.89,10.9 R9.P$2
N$13
  Bottom 0.254: J1.24 68.35,10.9 R8.P$2
N$14
  Bottom 0.254: J1.21 65.81,10.9 R7.P$2
N$15
  Bottom 0.254: J1.18 63.27,10.9 R6.P$2
N$16
  Bottom 0.254: R5.P$2 60.71,7.64 J1.15
N$17
  Bottom 0.254: J1.12 58.19,10.9 R4.P$2
N$18
  Bottom 0.254: R3.P$2 55.63,7.64 J1.9
N$19
  Bottom 0.254: R2.P$2 53.09,7.64 J1.6
N$20
  Bottom 0.254: R1.P$2 50.55,7.64 J1.3
N$21  (via drill 0.3)
  Bottom 0.508: R25.P$2 v13.08,11.68 R23.P$1
  pour Top (no thermals): 12.32,13.46 12.24,12.22 12.32,12.06 12.32,11.05 13.59,11.05 13.59,12.06 13.08,12.57 13.08,13.46
N$23  (via drill 0.3)
  Top 0.254: 93.9,11.13 v93.98,11.05 93.91,11.12 U4.10
  Bottom 0.254: C2.P$1 93.92,11.09 v93.98,11.05
N$24  (via drill 0.3)
  Top 0.254: U6.2 11.76,16.2 v12.06,16.51
  Bottom 0.254: R27.P$1 11.68,16.12 v12.06,16.51 12.06,17.27 11.42,17.91 R26.P$2
N$25  (via drill 0.3)
  Top 0.254: U4.20 94.41,17.07 v94.61,17.27
  Bottom 0.254: 94.48,17.28 v94.61,17.27 94.48,17.14 C4.P$1
  Bottom 0.381: C4.P$1
N$27  (via drill 0.3)
  Top 0.406: J2.P$1 12.57,20.5 | v13.08,19.05 13.34,19.05 13.59,18.8
  Top 0.508: J2.P$1 12.56,19.87 13.08,19.36 v13.08,19.05
  Bottom 0.381: R25.P$1 13.09,13.46 v13.84,13.46
  Bottom 0.483: C23.P$1 12.69,19.44 v13.08,19.05
  pour Top (no thermals): 12.24,14.61 13.21,14.61 13.46,14.35 13.46,13.21 13.59,13.08 14.22,13.08 14.35,13.21 14.35,18.8 14.1,19.05 12.83,19.05 12.83,16 12.57,15.75 12.24,15.75
N$28  (via drill 0.3)
  Top 0.381: U6.7 11.76,11.74 v11.81,11.68
  Bottom 0.508: R24.P$1 v11.81,11.68
N$30
  cutout Route2: 92.43,23.16 92.94,23.67 96.04,23.67 96.01,20.07 92.46,20.07
N$31
  cutout Route3 (rank 5, no thermals): 92.46,23.67 96.04,23.67 96.01,20.07 92.46,20.07
N$32  (via drill 0.3)
  Top 0.254: U6.5 10.09,13.16 9.65,13.16 9.63,13.18 9.12,13.18 9.02,13.08 8.71,13.08
  Bottom 0.508: L1.P$2 v8,11.94
  pour Top (no thermals): 10.64,12.19 10.64,13.41 7.39,13.41 7.39,11.35 8.61,11.35 8.61,12.75 10.29,12.75 10.29,12.19
N$36  (via drill 0.3)
  Top 0.381: U6.6 11.11,11.87 10.92,11.68
  Bottom 0.508: C26.P$1 v9.55,12.01 8.36,10.82 7.04,10.82 6.43,11.43 6.43,17.96 7.38,18.91 R26.P$1
  pour Top (no thermals): 10.79,11.81 10.92,11.94 11.3,11.94 11.3,11.68 10.67,11.05 9.14,11.05 9.02,11.18 9.02,12.45 9.91,12.45 9.91,11.94 10.03,11.81
N$38  (via drill 0.3)
  Top 0.254: U1.3 85.92,13.39 v86.16,13.16
  Bottom 0.254: R15.P$1 D1.C 86.36,12.95 v86.16,13.16
PPM-SBUS-PROT
  Bottom 0.254: 83.57,7.64 J1.42
  Bottom 0.508: 83.57,7.64 R14.P$2 83.57,7.62
PPM_INPUT  (via drill 0.3)
  Top 0.254: U1.2 85.27,13.34 v85.09,13.16
  Bottom 0.254: R14.P$1 D2.C 84.96,13.03 v85.09,13.16
PWM_CH0  (via drill 0.3)
  Top 0.254: U5.6 73.45,19.01 v73.53,19.05
  Bottom 0.254: R1.P$1 | v73.53,19.05 73.51,19.07 70.74,19.07 70.56,18.9 69.57,18.9 67.56,16.89 58.5,16.89 57.56,15.95 55.07,15.95 52.12,13.01 51.61,13.01 R1.P$1 | 50.49,11.89 R1.P$1
PWM_CH1  (via drill 0.3)
  Top 0.254: U5.7 71.39,18.36 v71.32,18.29
  Bottom 0.254: v71.32,18.29 69.72,18.29 67.82,16.38 58.85,16.38 57.86,15.39 55.78,15.39 53.09,12.7 R2.P$1
PWM_CH2  (via drill 0.3)
  Top 0.254: U5.8 73.48,17.71 v73.53,17.65
  Bottom 0.254: v73.53,17.65 69.98,17.65 68.2,15.93 59.23,15.93 57.66,14.35 56.01,14.35 55.63,13.97 R3.P$1
PWM_CH3  (via drill 0.3)
  Top 0.254: U5.9 71.36,17.06 v71.32,17.02
  Bottom 0.254: R4.P$1 59.56,11.94 60.33,12.7 61.34,12.7 63.25,14.55 67.69,14.55 70.1,17.02 v71.32,17.02
PWM_CH4  (via drill 0.3)
  Top 0.254: U5.10 73.43,16.41 v73.53,16.38
  Bottom 0.254: R5.P$1 61.64,11.93 62.18,12.47 64.06,12.47 64.44,12.85 66.83,12.85 70.23,16.38 v73.53,16.38
PWM_CH5  (via drill 0.3)
  Top 0.254: U5.11 71.36,15.76 v71.32,15.75
  Bottom 0.254: v71.32,15.75 70.36,15.75 67.08,12.45 65.08,12.45 64.6,11.97 63.29,11.97 R6.P$1
PWM_CH6  (via drill 0.3)
  Top 0.254: U5.12 v73.54,15.11 v73.53,15.11
  Bottom 0.254: v73.53,15.11 70.48,15.11 67.31,11.89 R7.P$1
PWM_CH7  (via drill 0.3)
  Top 0.254: U5.13 71.34,14.46 v71.32,14.45
  Bottom 0.254: R8.P$1 70.86,14.47 70.97,14.47 | 70.97,14.47 71.12,14.48 | 70.97,14.47 71.32,14.47 v71.32,14.45
PWM_CH8  (via drill 0.3)
  Top 0.254: U5.15 74.43,13.81 v74.4,13.84
  Bottom 0.254: R9.P$1 71.49,11.93 73.41,13.84 v74.4,13.84 74.42,13.84
PWM_CH9  (via drill 0.3)
  Top 0.254: U5.16 76.4,14.46 v76.35,14.5
  Bottom 0.254: R10.P$1 74.41,11.93 75.06,12.57 75.06,13.21 v76.35,14.5
PWM_CH10  (via drill 0.3)
  Top 0.254: U5.17 v79.75,15.11 v79.76,15.11
  Bottom 0.254: v79.75,15.11 v79.76,15.11 76.57,11.93 R11.P$1
PWM_CH11  (via drill 0.3)
  Top 0.254: U5.18 v80.76,15.76 v80.77,15.75
  Bottom 0.254: v80.77,15.75 80.77,14.73 78.49,12.45 R12.P$1
PWM_CH12  (via drill 0.3)
  Top 0.254: U5.19 79.73,16.41 v79.76,16.38
  Bottom 0.254: R13.P$1 81.03,14.1 81.53,14.61 81.53,15.88 80.9,16.51 79.88,16.51 v79.76,16.38
PWM_OE  (via drill 0.3)
  Top 0.254: 77,18.88 v76.96,18.92 77.05,19.01 U5.23
  Bottom 0.254: J6.23 42.16,2.54 43.43,3.81 45.09,3.81 48.13,6.86 48.13,8.76 49.02,9.65 49.02,13.08 51.52,15.58 52.81,15.58 54.36,17.12 57,17.12 57.78,17.91 66.04,17.91 66.8,18.67 66.8,20.7 67.56,21.46 70.26,21.46 70.81,20.9 72.29,20.9 72.64,21.26 73.89,21.26 74.27,20.88 74.27,20.09 75.44,18.92 v76.96,18.92
SAFETY  (via drill 0.3)
  Top 0.254: 20.83,20.48 J10.P$3 20.85,19.96 20.07,19.18 v20.07,19.05 20.07,18.67 18.41,17.02 18.41,14.25 19.71,12.95 19.71,11.15 23.62,7.24 31.5,7.24 J6.18
  Bottom 0.254: R33.P$1 20.06,19.18 v20.07,19.05
SB
  Bottom 0.508: J1.45 87.76,9.25 R15.P$2 87.76,9.27 86.11,7.62
SBUS_INPUT  (via drill 0.3)
  Top 0.254: U1.6 85.92,18.49 v85.98,18.54 86.11,18.67 87.88,18.67 TP2.TP
  Bottom 0.254: J6.25 44.96,2.54 49.02,6.6 49.02,8.64 49.66,9.27 49.66,12.83 51.37,14.54 52.59,14.54 54.61,16.56 57.3,16.56 58.14,17.4 67.31,17.4 69.34,19.43 69.34,20.07 69.83,20.55 70.31,20.55 71.04,19.81 73.79,19.81 74.3,19.3 74.3,18.26 74.95,17.6 85.04,17.6 v85.98,18.54
SBUS_OUTPUT  (via drill 0.3)
  Top 0.254: U1.5 86.57,17.14 v87.02,16.69 87.48,16.23 87.48,16.05 88.9,14.63 TP1.TP 86.74,12.45 84.71,12.45 81.79,9.53 48.39,9.53 45.72,6.86 45.72,2.21 44.91,1.4 35.26,1.4 34.92,1.73 34.92,3.3 36.2,4.57 J6.20
SPI_CLK  (via drill 0.3)
  Top 0.254: J5.P$2 66.13,19.09 v66.17,19.18 | v89.15,19.05 90.17,19.05 91.67,17.55 92.08,17.55 92.87,16.76 U4.23
  Bottom 0.254: J6.11 27.18,1.4 34.16,1.4 34.92,2.16 34.92,3.17 35.56,3.81 36.7,3.81 37.47,4.57 37.47,6.35 38.35,7.24 45.85,7.24 48.39,9.78 48.39,13.49 51.28,16.38 52.65,16.38 54,17.73 56.59,17.73 57.28,18.41 65.41,18.41 v66.17,19.18 66.17,21.46 67.26,22.55 71.32,22.55 72.08,21.79 74.19,21.79 74.8,21.18 74.8,20.45 75.69,19.56 78.23,19.56 79.63,20.95 80.42,20.95 81.48,22.02 81.48,22.45 82.27,23.24 85.22,23.24 87.88,20.57 88.59,20.57 89.15,20.02 v89.15,19.05
SPI_CS  (via drill 0.3)
  Top 0.254: v82.17,13.34 80.26,11.43 70.61,11.43 70.1,11.94 70.1,16.79 69.11,17.78 63.8,17.78 62.84,18.75 62.83,18.88 62.83,19.51 62.38,19.96 | v88.9,12.06 89.41,12.06 90.93,10.54 92.46,10.54 92.87,10.95 U4.8 | 62.36,20.47 62.38,20.45 J5.P$5 62.38,19.96 | 62.38,19.96 62.38,18.82 61.98,18.41 61.44,18.41 60.81,19.05 58.37,19.05 57.2,20.22 57.2,21.54 v57.15,21.59
  Bottom 0.254: J6.5 17.14,3.81 17.14,5.71 18.41,6.99 18.41,13.08 20.57,15.24 25.91,15.24 32.89,22.23 53.72,22.23 54.36,21.59 v57.15,21.59 | v88.9,12.06 87.12,13.82 84.3,13.82 83.82,13.34 v82.17,13.34
SPI_INT
  Top 0.254: J6.14 29.87,3.79 29.87,1.52 30.5,0.89 45.54,0.89 46.56,1.91 46.56,6.04 49.4,8.89 82.73,8.89 84.86,11.02 88.88,11.02 89.99,9.91 91.57,9.91 92.89,8.59 94.36,8.59 94.92,9.14 U4.12
SPI_MISO  (via drill 0.3)
  Top 0.254: J5.P$3 64.88,19.2 v64.9,19.18 | v93.22,9.27 93.22,10.56 93.37,10.71 U4.9
  Bottom 0.254: v64.9,19.18 64.9,19.05 | v64.9,19.18 65.41,19.68 65.41,22.17 66.73,23.5 71.2,23.5 72.31,22.38 74.47,22.38 75.39,21.46 75.39,20.75 76.07,20.07 77.85,20.07 79.38,21.59 80.29,21.59 80.85,22.15 80.85,22.61 82.12,23.88 85.85,23.88 86.36,23.37 86.87,23.37 89.79,20.45 89.79,11.79 92.33,9.25 93.19,9.25 v93.22,9.27 | J6.7 19.79,1.37 15.27,1.37 14.61,2.03 14.61,6.07 14.05,6.63 14.05,11.58 14.61,12.14 14.61,12.95 18.16,16.51 25.65,16.51 32,22.86 54.1,22.86 54.74,22.23 61.85,22.23 v64.9,19.18
SPI_MOSI  (via drill 0.3)
  Top 0.254: U4.24 92.36,16.45 92.08,16.74 90.81,16.74 90.42,16.36 90.42,13.97 89.53,13.08 v88.9,13.08 | J5.P$4 v63.63,19.05 64.26,18.41 69.85,18.41 70.61,17.65 70.61,12.45 71.12,11.94 79.63,11.94 v82.17,14.48
  Bottom 0.254: J6.9 24.64,3.81 26.54,3.81 27.3,4.57 27.3,5.97 27.81,6.48 30.35,6.48 33.15,9.27 44.45,9.27 46.23,11.05 46.23,15.49 45.59,16.13 45.59,20.07 47.12,21.59 53.47,21.59 54.1,20.95 61.72,20.95 v63.63,19.05 | v88.9,13.08 87.87,14.06 | 87.87,14.06 87.81,14.12 | v82.17,14.48 83.39,14.48 83.54,14.3 87.61,14.3 87.87,14.06
SPI_OE  (via drill 0.3)
  Top 0.254: J5.P$6 61.13,19.9 61.72,19.3 v61.72,19.05
  Bottom 0.254: J6.16 31.11,6.1 33.78,8.76 44.83,8.76 46.74,10.54 46.74,16.26 46.23,16.76 46.23,19.81 47.24,20.83 53.21,20.83 53.67,20.37 56.59,20.37 57.91,19.05 v61.72,19.05
UART1_CTS  (via drill 0.3)
  Top 0.254: J3.P$4 v39.38,11.44 v39.37,11.43
  Bottom 0.254: v39.38,11.44 v39.37,11.43 38.46,12.34 36.47,12.34 35.56,11.43 33.27,11.43 29.72,7.87 26.29,7.87 J6.10
UART1_RTS  (via drill 0.3)
  Top 0.254: J3.P$5 38.13,11.46 v38.1,11.43
  Bottom 0.254: J6.12 26.04,6.22 27.05,7.24 29.97,7.24 33.15,10.41 37.08,10.41 v38.1,11.43
UART1_RXD  (via drill 0.3)
  Top 0.254: J3.P$3 40.63,11.41 v40.64,11.43
  Bottom 0.254: J6.8 20.95,6.35 23.37,8.76 29.59,8.76 33.22,12.39 35.36,12.39 36.12,13.16 38.91,13.16 v40.64,11.43
UART1_TXD  (via drill 0.3)
  Top 0.254: J3.P$2 41.88,11.45 40.84,10.41 35.18,10.41 34.14,11.46 v34.14,13.31
  Bottom 0.254: J6.6 19.94,6.6 19.94,12.57 21.3,13.94 33.51,13.94 v34.14,13.31
UART2_RXD  (via drill 0.3)
  Top 0.254: J4.P$3 v35.42,19.19 v35.43,19.18 | J6.19 37.47,3.81 37.47,6.86 39.12,8.51 40.72,8.51 v42.09,9.88
  Bottom 0.254: v42.09,9.88 41.45,10.52 41.45,11.89 35.43,17.91 v35.43,19.18
UART2_TXD  (via drill 0.3)
  Top 0.254: J6.17 33.66,3.17 34.92,4.45 34.92,6.6 37.69,9.33 37.89,9.53 40.82,9.53 41.96,10.67 42.82,10.67 v43.18,10.36 | J4.P$2 36.67,19.21 v36.7,19.18
  Bottom 0.254: v43.18,10.36 42.11,11.43 42.11,12.88 36.7,18.29 v36.7,19.18
VCCIO
  pour Route3 (rank 5, no thermals): 1.14,14.22 5.97,14.22 5.97,10.41 52.45,10.41 55.5,7.37 69.6,7.37 72.64,10.41 84.71,10.41 84.71,1.14 1.14,1.02

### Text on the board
Top: PB, AM, DRONE-LURE FAB A | LAYER 1 (PRIMARY SIDE) | 1 | 1 | 4
Route2: PB, AM, DRONE-LURE FAB A | LAYER 2 (INTERNAL GND) | 2 | 2 | 4
Route3: PB, AM, DRONE-LURE FAB A | LAYER 3 (INTERNAL POWER) | 3 | 3 | 4
Bottom: PB# IC-DRONE-LURE-0001- | PB, AM, DRONE-LURE FAB A | LAYER 4 (SECONDARY SIDE) | 4 | 4 | 4 | 4
tPlace: 1 | 2
bPlace: 2 | 2
tNames: Buzzer | Safety | Telemetry2 | SPI | Alt / Pwr | PWR | GPS | ADC | Servo / Power | +5VSB | PB, AM, SS, DRONE-LURE FAB A, P | SILKSCREEN (PRIMARY SIDE)
bNames: PB, AM, SS, DRONE-LURE FAB A, S | SILKSCREEN (SECONDARY SIDE)
tStop: PB, AM, SM, DRONE-LURE FAB A, P | SOLDER MASK (PRIMARY)
bStop: PB, AM, SM, DRONE-LURE FAB A, S | SOLDER MASK (SECONDARY)
tCream: PBA, AM, SP, DRONE-LURE FAB A, P | SOLDER PASTE (PRIMARY)
bCream: PBA, AM, SP, DRONE-LURE FAB A, S | SOLDER PASTE (SECONDARY)
Reference: Released under the Creative Commons Attribution Share-Alike 3.0 License / http://creativecommons.org/licenses/by-sa/3.0
_tsilk: ASSEMBLY PRIMARY SIDE
_bsilk: ASSEMBLY SECONDARY SIDE
DrillLegend: LAYER-STACK | 10
Panel: 2
FAB_NOTES: LAYER STACKUP | LAYER 1 - 0.5 Oz.Cu. | PRPREG (~.0037") | LAYER 2 - 1.0 Oz.Cu. | CORE (~.0490") | LAYER 3 - 1.0 Oz.Cu. | PRPREG (~.0037") | LAYER 4 - 0.5 Oz.Cu. | FINISHED BOARD THICKNESS TO BE .062 +.008"-.005" | NOTES: UNLESS OTHERWISE SPECIFIED: / 1. PART NUMBER IS PARENT ITEM IDENTIFICATION NUMBER ON / ENGINEERING BILL OF MATERIAL. / 2. THIS DRAWING ALSO EXISTS ON ELECTRONIC MEDIA. / 3. FABRICATE PER INTEL SPECIFICATION A84501 LATEST REVISION. / 4. THE CENTER OF THIS HOLE WILL ESTABLISH DATUM -B-. / 5. DATUM -A- IS ESTABLISHED PERPENDICULAR TO DATUM -B- THROUGH / THE CENTER OF THIS HOLE. / 6. DIMENSIONING AND TOLERANCING PER ANSI Y14.5M. / 7. ALL CONTROLLED IMPEDANCE IS +/- 15%. / 8. SOLDERMASK COLOR TO BE GREEN WITH WHITE SILKSCREEN. / 9. SURFACE FINISH: PLATE ENIG PER INTEL PCB SPECIFICATION A84501 / 10. SIZES SPECIFIED ARE FINISHED HOLE SIZE / 11. FINISHED BOARD MUST BE COMPLIANT WITH THE RESTRICTION ON USE OF HAZARDOUS / SUBSTANCES (RoHS) DIRECTIVE. TEST DATA MUST BE AVAILABLE TO DEMONSTRATE / THAT IT WILL BE ABLE TO RELIABLY HANDLE REPEATED EXPOSURE TO ELEVATED / TEMPERATURES REQUIRED ON LEAD FREE SOLDER PROCESS. / A. A RoHS COMPLIANCE CERTIFICATE SHALL BE AVAILABLE UPON REQUEST / B. THE LEAD FREE AND "e1" SOLDER CATEGORY MARKS MUST BE ADDED TO THE SILKSCREEN / C. THE BOARD PACKAGE MUST BE IDENTIFIED AS RoHS COMPLIANT. PACKAGE OF / FINISHED PANELS MUST BE IDENTIFIED AS RoHS COMPLIANT. / 12. VENDOR SHALL RECEIVE STACK-UP APPROVAL PRIOR TO FAB START. / 13. MAXIMUM SOLDERMASK OFFSET TO BE 3 MILS. / 14. FABRICATION VENDOR TO MARK DASH NUMBER OF / PART NUMBER APPROXIMATELY WHERE SHOWN ON SECONDARY SIDE. / 15. IDENTIFICATION NUMBER PER INTEL MARKING STANDARDS / 16. PCB MATERIAL: FR4 | 1
Multi_Layer: MASTER | 04-14-15 | TITLE | SHEET | TITLE | REV | SCALE 1:1 | LAYER | DOCUMENT NUMBER | S | IC-DRONE-LURE-0001 | A1 | SHEET | OF
LOGO_OUTLINE: ADN | 04-14-15 | CNG | 04-14-15 | JOHNX L | 04-14-15 | PB,FAB DRAWING / DRONE-LURE | IC-DRONE-LURE-0001 | A1 | SHEET | OF | 2

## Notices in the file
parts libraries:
SparkFun-DigitalIC: Licensing: Creative Commons ShareAlike 4.0 International - https://creativecommons.org/licenses/by-sa/4.0
